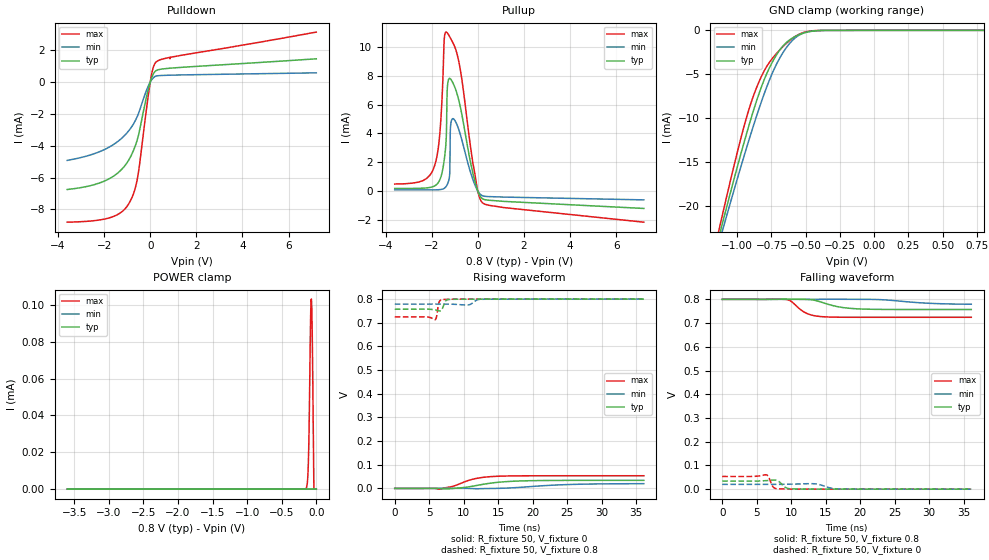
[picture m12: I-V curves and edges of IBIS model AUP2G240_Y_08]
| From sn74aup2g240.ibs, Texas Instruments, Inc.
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[Model]   AUP2G240_Y_08
Model_type  3-state
Enable   Active-Low
Vref =   0
Rref =   1E6
Cref =   30p
Vmeas =   0.4
| variable   typ   min   max
C_comp   2.23pF   2.10pF   2.51pF
| C_pullup   2.65pF   2.24pF   3.06pF
| C_pulldown   2.53pF   2.22pF   2.84pF
| C_tri-state   2.23pF   2.10pF   2.51pF
[Temperature Range]   40   100   -40
| Ambient temperature   25   85   -40
[Voltage range]   0.8   0.8   0.8
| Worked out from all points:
|   slope of the pulldown table from 0 to 0.12 V, typ, clamps not added: 257 ohm
|   slope of the pullup table from 0 to 0.12 V, typ, clamps not added: 311 ohm
|   GND clamp passes 1 mA (typ) near -0.61 V on its own axis
[GND Clamp]
| AUP2G240_Y_08
|   Voltage   I(typ)   I(min)   I(max)
-3.6V     -191.7mA   -177.9mA   -208.5mA
-1.13V    -23.31mA   -24.02mA   -22.49mA
-1.11V    -22.09mA   -22.91mA   -21.13mA
-1.09V    -20.88mA   -21.8mA    -19.78mA
-970mV    -13.87mA   -15.34mA   -12.08mA
-870mV    -8.57mA    -10.3mA    -6.977mA
-755mV    -3.961mA   -5.291mA   -3.435mA
-685mV    -2.151mA   -3.036mA   -2.16mA
-625mV    -1.183mA   -1.642mA   -1.265mA
-530mV    -386.3uA   -402uA     -324.2uA
-420mV    -46.16uA   -47.89uA   -21.13uA
800mV     102.8pA    541pA      15.75pA
[POWER Clamp]
| AUP2G240_Y_08
|   Voltage   I(typ)   I(min)   I(max)
-3.6V     1.402nA    2.9nA      449.8pA
-155mV    816.4pA    3.701nA    159.7nA
-130mV    2.826nA    7.394nA    3.34uA
-115mV    8.067nA    11.11nA    14.03uA
-105mV    15.97nA    13.72nA    31.02uA
-85mV     40.58nA    14.86nA    86.89uA
-80mV     43.57nA    13.98nA    97.29uA
-70mV     38.76nA    11.17nA    103.2uA
-65mV     31.78nA    9.496nA    98.04uA
-55mV     15.85nA    6.291nA    73.51uA
-35mV     1.046nA    2.306nA    21.47pA
0V        0A         0A         0A
[Pulldown]
| AUP2G240_Y_08
|   Voltage   I(typ)   I(min)   I(max)
-3.6V     -6.749mA   -4.919mA   -8.802mA
-1.86V    -6.133mA   -4.148mA   -8.564mA
-1.27V    -5.529mA   -3.571mA   -8.188mA
-895mV    -4.804mA   -2.991mA   -7.55mA
-705mV    -4.217mA   -2.575mA   -6.921mA
-565mV    -3.63mA    -2.167mA   -6.118mA
-470mV    -3.08mA    -1.812mA   -5.243mA
-155mV    -882uA     -491.6uA   -1.594mA
15mV      70.31uA    36.95uA    134.1uA
140mV     523.3uA    274.6uA    953.9uA
280mV     740uA      385.5uA    1.291mA
7.2V      1.459mA    578.6uA    3.138mA
[Pullup]
| AUP2G240_Y_08
|   Voltage   I(typ)   I(min)   I(max)
-3.6V     178.6uA    77.27uA    485.5uA
-1.88V    346.9uA    79.15uA    1.719mA
-1.645V   779.6uA    96.46uA    3.979mA
-1.455V   2.149mA    186.2uA    10.49mA
-1.37V    3.579mA    320.8uA    11.05mA
-1.3V     7.498mA    532.5uA    10.95mA
-1.215V   7.833mA    1.212mA    10.72mA
-1.18V    7.79mA     4.496mA    10.62mA
-1.07V    7.494mA    5.036mA    10.29mA
0V        0A         0A         0A
200mV     -531.6uA   -328.5uA   -817.8uA
7.2V      -1.213mA   -616.6uA   -2.168mA
[Ramp]
| AUP2G240_Y_08
| variable   typ   min   max
dV/dt_r   0.02/5.01E-09   0.01/7.31E-09   0.03/3.50E-09
dV/dt_f   0.03/3.48E-09   0.01/5.60E-09   0.05/2.10E-09
R_load = 50
[Rising Waveform]
| AUP2G240_Y_08
R_fixture =   50
C_fixture =   0
L_fixture =   0
V_fixture =   0
V_fixture_min = 0
V_fixture_max = 0
|   Time   V(typ)   V(min)   V(max)
0s        5.542nV    24.01nV    351.9pV
5.757ns   166.5uV    -4.182uV   162.8uV
6.557ns   4.573uV    -1.554uV   -2.998mV
7.389ns   -2.277mV   18.79uV    2.978mV
8.565ns   75.42uV    95.39uV    10.06mV
11.53ns   10.51mV    -1.109mV   40.29mV
14.46ns   24.19mV    -144.3uV   50.67mV
18.51ns   31.75mV    5.171mV    53.18mV
25.13ns   33.86mV    16.28mV    53.49mV
36.1ns    34.06mV    20.01mV    53.5mV
[Falling Waveform]
| AUP2G240_Y_08
R_fixture =   50
C_fixture =   0
L_fixture =   0
V_fixture =   0.8
V_fixture_min = 0.8
V_fixture_max = 0.8
|   Time   V(typ)   V(min)   V(max)
0s        800mV      800mV      800mV
9.381ns   800.8mV    800mV      798.9mV
9.989ns   800.5mV    799.9mV    791.4mV
11.35ns   800.2mV    799.9mV    756.8mV
12.19ns   799.8mV    799.9mV    741.7mV
14.66ns   785.4mV    800.4mV    726.6mV
17.03ns   767.6mV    800.4mV    724.7mV
19.83ns   759.7mV    800.1mV    724.4mV
30.28ns   757.2mV    783mV      724.4mV
36.1ns    757.1mV    779.3mV    724.4mV
[Rising Waveform]
| AUP2G240_Y_08
R_fixture =   50
C_fixture =   0
L_fixture =   0
V_fixture =   0.8
V_fixture_min = 0.8
V_fixture_max = 0.8
|   Time   V(typ)   V(min)   V(max)
0s        757.1mV    778.6mV    724.4mV
5.853ns   753.9mV    778.7mV    712.5mV
6.053ns   752.6mV    778.7mV    724.8mV
6.437ns   750mV      778.8mV    787.4mV
7.093ns   773.5mV    778.8mV    798.4mV
7.477ns   795mV      778.7mV    798.8mV
8.205ns   798.8mV    778.3mV    799.3mV
10.68ns   799.6mV    775.2mV    799.8mV
12.52ns   799.8mV    798.9mV    799.9mV
36.1ns    800mV      800mV      800mV
[Falling Waveform]
| AUP2G240_Y_08
R_fixture =   50
C_fixture =   0
L_fixture =   0
V_fixture =   0
V_fixture_min = 0
V_fixture_max = 0
|   Time   V(typ)   V(min)   V(max)
0s        34.06mV    20.29mV    53.5mV
6.357ns   35.96mV    20.17mV    60.6mV
6.693ns   36.69mV    20.17mV    52.43mV
7.405ns   38.51mV    20.19mV    8.608mV
8.061ns   34.97mV    20.29mV    1.636mV
9.189ns   7.134mV    20.7mV     636.3uV
10.03ns   1.216mV    21.18mV    405.4uV
13.45ns   305.5uV    22.42mV    23.55uV
16.97ns   64.4uV     854.5uV    1.26uV
36.1ns    79.49nV    8.183uV    35.37nV
